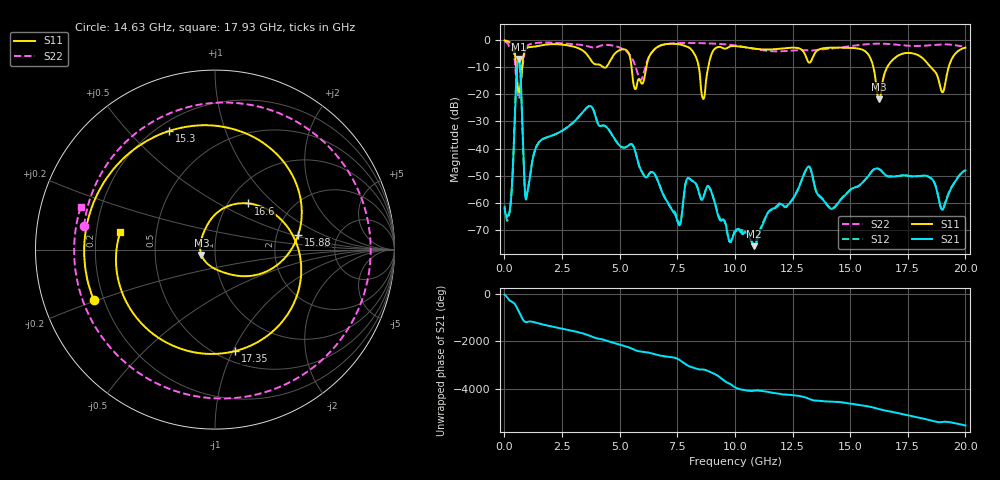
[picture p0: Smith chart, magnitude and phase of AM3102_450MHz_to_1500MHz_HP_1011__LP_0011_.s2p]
!Agilent Technologies,E8364B,MY43040894,A.07.50.67
!Agilent E8364B: A.07.50.67
!Date: Thursday, January 11, 2018 06:23:39
!Correction: S11(Full 2 Port(1,2))
!S21(Full 2 Port(1,2))
!S12(Full 2 Port(1,2))
!S22(Full 2 Port(1,2))
!S2P File: Measurements: S11, S21, S12, S22:
# Hz S  dB  R 50
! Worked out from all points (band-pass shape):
!   1601 points, 10 MHz to 20 GHz, reference 50 ohm
!   highest |S21| = -6.90 dB at 622.2 MHz (marker M1); lowest = -76.1 dB at 10.84 GHz (marker M2)
!   |S21| within 3 dB of the highest: 557.9 MHz to 681.6 MHz (123.7 MHz wide, 20 % of centre)
!   lowest |S11| = -21.8 dB at 16.25 GHz (marker M3), VSWR 1.18, Z = 42.9 - j2.61 ohm
!   |S11| at or under -10 dB: 5.52 GHz to 6.156 GHz (636.4 MHz wide, 10.9 % of centre); 16.01 GHz to 16.6 GHz (592.1 MHz wide, 3.63 % of centre); 18.5 GHz to 19.27 GHz (767.9 MHz wide, 4.07 % of centre)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
!   |S22| runs from -21.5 to -0.4 dB; largest |S21 - S12| = 0.0018
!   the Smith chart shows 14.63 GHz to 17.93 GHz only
!   S11 on the Smith chart (normalised r, x): 14.63 GHz: 0.16, -0.19; 15.3 GHz: 0.25, +0.66; 15.88 GHz: 2.64, +0.54; 16.6 GHz: 1.23, +0.70; 17.35 GHz: 0.60, -1.02; 17.93 GHz: 0.30, +0.08
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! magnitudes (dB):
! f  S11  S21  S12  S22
! 10 MHz  -0.1  -62.2  -61.1  -0.4
! 259.9 MHz  -0.9  -61.1  -61.1  -3.1
! 622.2 MHz  -18.9  -6.9  -6.9  -21.5
! 972 MHz  -2.8  -57.4  -57.2  -2.2
! 3.346 GHz  -3.5  -27.1  -27.1  -1.7
! 5.682 GHz  -18.1  -41.1  -41.2  -9.5
! 6.682 GHz  -2.2  -52.5  -52.4  -2.4
! 7.569 GHz  -1.5  -68.2  -67.5  -1.0
! 8.618 GHz  -21.6  -58.4  -58.3  -1.1
! 10.01 GHz  -2.1  -70.7  -70.9  -1.9
! 10.84 GHz  -3.1  -76.1  -75.1  -3.1
! 13.34 GHz  -7.1  -49.3  -49.2  -3.8
! 14.63 GHz  -2.7  -58.6  -58.4  -2.6
! 15.3 GHz  -3.0  -54.2  -54.0  -1.8
! 15.88 GHz  -6.6  -49.1  -49.1  -1.3
! 16.25 GHz  -21.8  -47.6  -47.5  -1.2
! 16.6 GHz  -10.0  -50.2  -50.2  -1.3
! 16.68 GHz  -9.0  -50.3  -50.3  -1.4
! 17.35 GHz  -4.8  -49.9  -49.9  -1.9
! 17.93 GHz  -5.4  -50.2  -50.2  -2.1
! 19.01 GHz  -19.2  -62.6  -62.2  -1.5
! 20 GHz  -2.7  -48.1  -48.1  -2.4
